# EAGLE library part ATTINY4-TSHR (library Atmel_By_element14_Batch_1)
Microcontroller
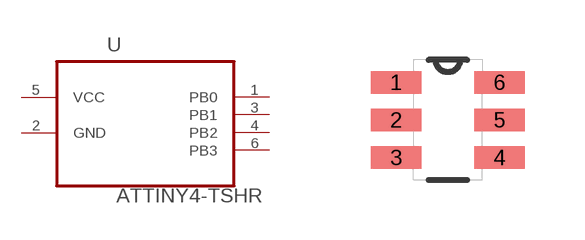
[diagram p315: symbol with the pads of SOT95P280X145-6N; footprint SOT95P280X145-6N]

Designator prefix U

## ATTINY4-TSHR (DESCRIPTION: Microcontroller; MPN: ATTINY4-TSHR; OC_FARNELL: 1841625; OC_NEWARK: 12T1337; PACKAGE: SOT563-6; SUPPLIER: ATMEL)  [SOT95P280X145-6N]
1  PB0
2  GND  pas
3  PB1
4  PB2
5  VCC  pwr
6  PB3

## Footprint SOT95P280X145-6N (pad centres in mm)
smd 1.27 x 0.559: 1 -1.295,0.94; 2 -1.295,0; 3 -1.295,-0.94; 4 1.295,-0.94; 5 1.295,0; 6 1.295,0.94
